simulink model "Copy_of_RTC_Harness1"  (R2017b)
settings: Solver=FixedStepDiscrete  StartTime=0.0  StopTime=4  FixedStep=0.01  RelTol=1e-3  EnableMultiTasking=on
undefined symbols (not defined in the file): sigbuilder_block

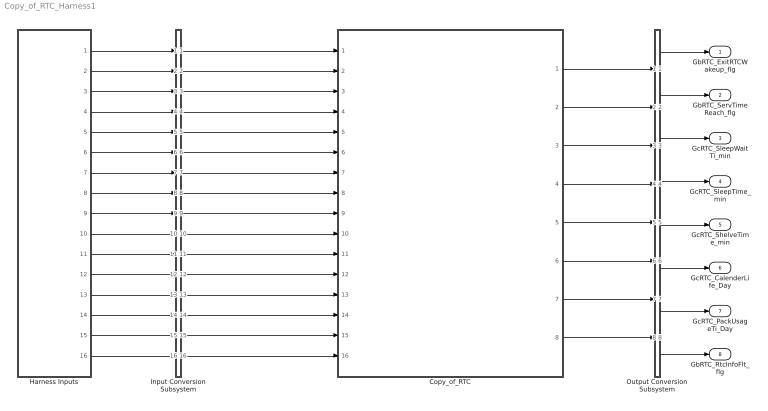
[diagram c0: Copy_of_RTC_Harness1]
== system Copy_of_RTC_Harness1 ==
  Copy_of_RTC : ModelReference  ModelNameDialog=Copy_of_RTC  SimulationMode=Normal  ModelReferenceVersion='M101C100'
  Harness Inputs : Subsystem  Tag=STV Subsys  LoadFcn=sigbuilder_block('load');  StartFcn=sigbuilder_block('start');  StopFcn=sigbuilder_block('stop');  ClipboardFcn=sigbuilder_block('clipboard');  mask(Sigbuilder block){tuvar=[0:10]}
      mask init:
      | if ~strcmp(get_param(bdroot(gcb),'SimulationStatus'),'stopped'),tuvar = sigbuilder_block('maskInit'); end
  Input Conversion Subsystem : Subsystem  Tag=__SLT_ICS__  Description=Signal spec. and routing
  Output Conversion Subsystem : Subsystem  Tag=__SLT_OCS__  Description=Signal spec. and routing
  GbRTC_ExitRTCWakeup_flg : Outport  OutDataTypeStr=boolean  PortDimensions=[1]
  GbRTC_ServTimeReach_flg : Outport  Port=2  OutDataTypeStr=boolean  PortDimensions=[1]
  GcRTC_SleepWaitTi_min : Outport  Port=3  OutDataTypeStr=uint16  PortDimensions=[1]
  GcRTC_SleepTime_min : Outport  Port=4  OutDataTypeStr=uint32  PortDimensions=[1]
  GcRTC_ShelveTime_min : Outport  Port=5  OutDataTypeStr=uint32  PortDimensions=[1]
  GcRTC_CalenderLife_Day : Outport  Port=6  OutDataTypeStr=uint32  PortDimensions=[1]
  GcRTC_PackUsageTi_Day : Outport  Port=7  OutDataTypeStr=uint32  PortDimensions=[1]
  GbRTC_RtcInfoFlt_flg : Outport  Port=8  OutDataTypeStr=boolean  PortDimensions=[1]
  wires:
  Harness Inputs/1(GbADP_RealTimeVld_flg) -> Input Conversion Subsystem/1(Inport_1)
  Harness Inputs/2(GbNDP_ReadShutdownTimeVld_flg) -> Input Conversion Subsystem/2(Inport_2)
  Harness Inputs/3(GcADP_YearSet_Yr) -> Input Conversion Subsystem/3(Inport_3)
  Harness Inputs/4(GcADP_MonthSet_Mn) -> Input Conversion Subsystem/4(Inport_4)
  Harness Inputs/5(GcADP_DaySet_D) -> Input Conversion Subsystem/5(Inport_5)
  Harness Inputs/6(GcADP_HourSet_Hr) -> Input Conversion Subsystem/6(Inport_6)
  Harness Inputs/7(GcADP_MinSet_Min) -> Input Conversion Subsystem/7(Inport_7)
  Harness Inputs/8(GcADP_SecondSet_S) -> Input Conversion Subsystem/8(Inport_8)
  Harness Inputs/9(GcISP_EcuOffTi_s) -> Input Conversion Subsystem/9(Inport_9)
  Harness Inputs/10(GeISP_EcuOffTiSt_enum) -> Input Conversion Subsystem/10(Inport_10)
  Harness Inputs/11(GeADP_AppChrgOrdCmd_enum) -> Input Conversion Subsystem/11(Inport_11)
  Harness Inputs/12(GeADP_AppChrgOrdStart_enum) -> Input Conversion Subsystem/12(Inport_12)
  Harness Inputs/13(GeMSM_BMUState_enum) -> Input Conversion Subsystem/13(Inport_13)
  Harness Inputs/14(GeODP_ObcCcSt_enum) -> Input Conversion Subsystem/14(Inport_14)
  Harness Inputs/15(GcADP_AcmDist_numb) -> Input Conversion Subsystem/15(Inport_15)
  Harness Inputs/16(GeCTC_CtrCtlState_enum) -> Input Conversion Subsystem/16(Inport_16)
  Output Conversion Subsystem/1(Outport_1) -> GbRTC_ExitRTCWakeup_flg/1
  Output Conversion Subsystem/2(Outport_2) -> GbRTC_ServTimeReach_flg/1
  Output Conversion Subsystem/3(Outport_3) -> GcRTC_SleepWaitTi_min/1
  Output Conversion Subsystem/4(Outport_4) -> GcRTC_SleepTime_min/1
  Output Conversion Subsystem/5(Outport_5) -> GcRTC_ShelveTime_min/1
  Output Conversion Subsystem/6(Outport_6) -> GcRTC_CalenderLife_Day/1
  Output Conversion Subsystem/7(Outport_7) -> GcRTC_PackUsageTi_Day/1
  Output Conversion Subsystem/8(Outport_8) -> GbRTC_RtcInfoFlt_flg/1
  Input Conversion Subsystem/1(Outport_1) -> Copy_of_RTC/1
  Input Conversion Subsystem/2(Outport_2) -> Copy_of_RTC/2
  Input Conversion Subsystem/3(Outport_3) -> Copy_of_RTC/3
  Input Conversion Subsystem/4(Outport_4) -> Copy_of_RTC/4
  Input Conversion Subsystem/5(Outport_5) -> Copy_of_RTC/5
  Input Conversion Subsystem/6(Outport_6) -> Copy_of_RTC/6
  Input Conversion Subsystem/7(Outport_7) -> Copy_of_RTC/7
  Input Conversion Subsystem/8(Outport_8) -> Copy_of_RTC/8
  Input Conversion Subsystem/9(Outport_9) -> Copy_of_RTC/9
  Input Conversion Subsystem/10(Outport_10) -> Copy_of_RTC/10
  Input Conversion Subsystem/11(Outport_11) -> Copy_of_RTC/11
  Input Conversion Subsystem/12(Outport_12) -> Copy_of_RTC/12
  Input Conversion Subsystem/13(Outport_13) -> Copy_of_RTC/13
  Input Conversion Subsystem/14(Outport_14) -> Copy_of_RTC/14
  Input Conversion Subsystem/15(Outport_15) -> Copy_of_RTC/15
  Input Conversion Subsystem/16(Outport_16) -> Copy_of_RTC/16
  Copy_of_RTC/1 -> Output Conversion Subsystem/1(Inport_1)
  Copy_of_RTC/2 -> Output Conversion Subsystem/2(Inport_2)
  Copy_of_RTC/3 -> Output Conversion Subsystem/3(Inport_3)
  Copy_of_RTC/4 -> Output Conversion Subsystem/4(Inport_4)
  Copy_of_RTC/5 -> Output Conversion Subsystem/5(Inport_5)
  Copy_of_RTC/6 -> Output Conversion Subsystem/6(Inport_6)
  Copy_of_RTC/7 -> Output Conversion Subsystem/7(Inport_7)
  Copy_of_RTC/8 -> Output Conversion Subsystem/8(Inport_8)

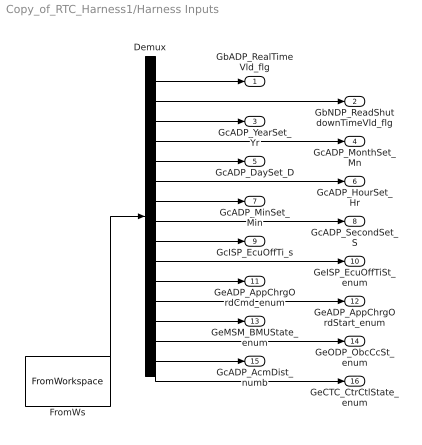
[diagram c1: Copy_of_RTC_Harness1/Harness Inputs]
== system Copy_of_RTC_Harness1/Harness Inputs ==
  Demux : Demux  Tag=STV Demux  Outputs=16
  FromWs : FromWorkspace  Tag=STV FromWs  VariableName=tuvar  SampleTime=0
  GbADP_RealTimeVld_flg : Outport  Tag=STV Outport
  GbNDP_ReadShutdownTimeVld_flg : Outport  Tag=STV Outport  Port=2
  GcADP_YearSet_Yr : Outport  Tag=STV Outport  Port=3
  GcADP_MonthSet_Mn : Outport  Tag=STV Outport  Port=4
  GcADP_DaySet_D : Outport  Tag=STV Outport  Port=5
  GcADP_HourSet_Hr : Outport  Tag=STV Outport  Port=6
  GcADP_MinSet_Min : Outport  Tag=STV Outport  Port=7
  GcADP_SecondSet_S : Outport  Tag=STV Outport  Port=8
  GcISP_EcuOffTi_s : Outport  Tag=STV Outport  Port=9
  GeISP_EcuOffTiSt_enum : Outport  Tag=STV Outport  Port=10
  GeADP_AppChrgOrdCmd_enum : Outport  Tag=STV Outport  Port=11
  GeADP_AppChrgOrdStart_enum : Outport  Tag=STV Outport  Port=12
  GeMSM_BMUState_enum : Outport  Tag=STV Outport  Port=13
  GeODP_ObcCcSt_enum : Outport  Tag=STV Outport  Port=14
  GcADP_AcmDist_numb : Outport  Tag=STV Outport  Port=15
  GeCTC_CtrCtlState_enum : Outport  Tag=STV Outport  Port=16
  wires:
  FromWs/1 -> Demux/1
  Demux/1 -> GbADP_RealTimeVld_flg/1
  Demux/2 -> GbNDP_ReadShutdownTimeVld_flg/1
  Demux/3 -> GcADP_YearSet_Yr/1
  Demux/4 -> GcADP_MonthSet_Mn/1
  Demux/5 -> GcADP_DaySet_D/1
  Demux/6 -> GcADP_HourSet_Hr/1
  Demux/7 -> GcADP_MinSet_Min/1
  Demux/8 -> GcADP_SecondSet_S/1
  Demux/9 -> GcISP_EcuOffTi_s/1
  Demux/10 -> GeISP_EcuOffTiSt_enum/1
  Demux/11 -> GeADP_AppChrgOrdCmd_enum/1
  Demux/12 -> GeADP_AppChrgOrdStart_enum/1
  Demux/13 -> GeMSM_BMUState_enum/1
  Demux/14 -> GeODP_ObcCcSt_enum/1
  Demux/15 -> GcADP_AcmDist_numb/1
  Demux/16 -> GeCTC_CtrCtlState_enum/1

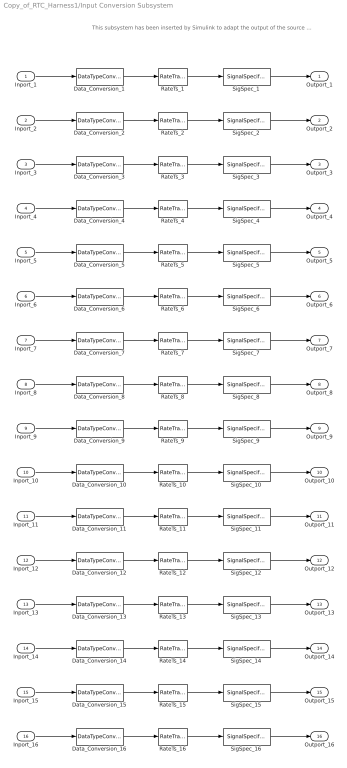
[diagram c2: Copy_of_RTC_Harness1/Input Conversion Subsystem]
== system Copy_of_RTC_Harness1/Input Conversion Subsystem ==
  note: This subsystem has been inserted by Simulink to adapt the output of the source blocks to the interface required by the harnessed component. Modifying the contents of this subsystem may result in compilation and simulation failure.
  Inport_1 : Inport
  Inport_2 : Inport  Port=2
  Inport_3 : Inport  Port=3
  Inport_4 : Inport  Port=4
  Inport_5 : Inport  Port=5
  Inport_6 : Inport  Port=6
  Inport_7 : Inport  Port=7
  Inport_8 : Inport  Port=8
  Inport_9 : Inport  Port=9
  Inport_10 : Inport  Port=10
  Inport_11 : Inport  Port=11
  Inport_12 : Inport  Port=12
  Inport_13 : Inport  Port=13
  Inport_14 : Inport  Port=14
  Inport_15 : Inport  Port=15
  Inport_16 : Inport  Port=16
  Data_Conversion_1 : DataTypeConversion  OutDataTypeStr=boolean
  Data_Conversion_{4..8,10..14,16} (11 alike) : DataTypeConversion  OutDataTypeStr=uint8
  Data_Conversion_15 : DataTypeConversion  OutDataTypeStr=single
  Data_Conversion_2 : DataTypeConversion  OutDataTypeStr=boolean
  Data_Conversion_3 : DataTypeConversion  OutDataTypeStr=uint16
  Data_Conversion_9 : DataTypeConversion  OutDataTypeStr=uint32
  RateTs_{1..16} (16 alike) : RateTransition  OutPortSampleTime=0.01
  SigSpec_1 : SignalSpecification  OutDataTypeStr=boolean  Unit=flg  Dimensions=[1]  SampleTime=0.01
  SigSpec_{10..13,16} (5 alike) : SignalSpecification  OutDataTypeStr=uint8  Unit=enum  Dimensions=[1]  SampleTime=0.01
  SigSpec_14 : SignalSpecification  OutDataTypeStr=uint8  Unit=numb  Dimensions=[1]  SampleTime=0.01
  SigSpec_15 : SignalSpecification  OutDataTypeStr=single  Unit=numb  Dimensions=[1]  SampleTime=0.01
  SigSpec_2 : SignalSpecification  OutDataTypeStr=boolean  Unit=flag  Dimensions=[1]  SampleTime=0.01
  SigSpec_3 : SignalSpecification  OutDataTypeStr=uint16  Unit=Yr  Dimensions=[1]  SampleTime=0.01
  SigSpec_4 : SignalSpecification  OutDataTypeStr=uint8  Unit=Min  Dimensions=[1]  SampleTime=0.01
  SigSpec_5 : SignalSpecification  OutDataTypeStr=uint8  Unit=Day  Dimensions=[1]  SampleTime=0.01
  SigSpec_6 : SignalSpecification  OutDataTypeStr=uint8  Unit=Hour  Dimensions=[1]  SampleTime=0.01
  SigSpec_7 : SignalSpecification  OutDataTypeStr=uint8  Unit=Min  Dimensions=[1]  SampleTime=0.01
  SigSpec_8 : SignalSpecification  OutDataTypeStr=uint8  Unit=S  Dimensions=[1]  SampleTime=0.01
  SigSpec_9 : SignalSpecification  OutDataTypeStr=uint32  Unit=s  Dimensions=[1]  SampleTime=0.01
  Outport_1 : Outport
  Outport_2 : Outport  Port=2
  Outport_3 : Outport  Port=3
  Outport_4 : Outport  Port=4
  Outport_5 : Outport  Port=5
  Outport_6 : Outport  Port=6
  Outport_7 : Outport  Port=7
  Outport_8 : Outport  Port=8
  Outport_9 : Outport  Port=9
  Outport_10 : Outport  Port=10
  Outport_11 : Outport  Port=11
  Outport_12 : Outport  Port=12
  Outport_13 : Outport  Port=13
  Outport_14 : Outport  Port=14
  Outport_15 : Outport  Port=15
  Outport_16 : Outport  Port=16
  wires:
  SigSpec_1/1 -> Outport_1/1
  RateTs_1/1 -> SigSpec_1/1
  Data_Conversion_1/1 -> RateTs_1/1
  Inport_1/1 -> Data_Conversion_1/1
  SigSpec_2/1 -> Outport_2/1
  RateTs_2/1 -> SigSpec_2/1
  Data_Conversion_2/1 -> RateTs_2/1
  Inport_2/1 -> Data_Conversion_2/1
  SigSpec_3/1 -> Outport_3/1
  RateTs_3/1 -> SigSpec_3/1
  Data_Conversion_3/1 -> RateTs_3/1
  Inport_3/1 -> Data_Conversion_3/1
  SigSpec_4/1 -> Outport_4/1
  RateTs_4/1 -> SigSpec_4/1
  Data_Conversion_4/1 -> RateTs_4/1
  Inport_4/1 -> Data_Conversion_4/1
  SigSpec_5/1 -> Outport_5/1
  RateTs_5/1 -> SigSpec_5/1
  Data_Conversion_5/1 -> RateTs_5/1
  Inport_5/1 -> Data_Conversion_5/1
  SigSpec_6/1 -> Outport_6/1
  RateTs_6/1 -> SigSpec_6/1
  Data_Conversion_6/1 -> RateTs_6/1
  Inport_6/1 -> Data_Conversion_6/1
  SigSpec_7/1 -> Outport_7/1
  RateTs_7/1 -> SigSpec_7/1
  Data_Conversion_7/1 -> RateTs_7/1
  Inport_7/1 -> Data_Conversion_7/1
  SigSpec_8/1 -> Outport_8/1
  RateTs_8/1 -> SigSpec_8/1
  Data_Conversion_8/1 -> RateTs_8/1
  Inport_8/1 -> Data_Conversion_8/1
  SigSpec_9/1 -> Outport_9/1
  RateTs_9/1 -> SigSpec_9/1
  Data_Conversion_9/1 -> RateTs_9/1
  Inport_9/1 -> Data_Conversion_9/1
  SigSpec_10/1 -> Outport_10/1
  RateTs_10/1 -> SigSpec_10/1
  Data_Conversion_10/1 -> RateTs_10/1
  Inport_10/1 -> Data_Conversion_10/1
  SigSpec_11/1 -> Outport_11/1
  RateTs_11/1 -> SigSpec_11/1
  Data_Conversion_11/1 -> RateTs_11/1
  Inport_11/1 -> Data_Conversion_11/1
  SigSpec_12/1 -> Outport_12/1
  RateTs_12/1 -> SigSpec_12/1
  Data_Conversion_12/1 -> RateTs_12/1
  Inport_12/1 -> Data_Conversion_12/1
  SigSpec_13/1 -> Outport_13/1
  RateTs_13/1 -> SigSpec_13/1
  Data_Conversion_13/1 -> RateTs_13/1
  Inport_13/1 -> Data_Conversion_13/1
  SigSpec_14/1 -> Outport_14/1
  RateTs_14/1 -> SigSpec_14/1
  Data_Conversion_14/1 -> RateTs_14/1
  Inport_14/1 -> Data_Conversion_14/1
  SigSpec_15/1 -> Outport_15/1
  RateTs_15/1 -> SigSpec_15/1
  Data_Conversion_15/1 -> RateTs_15/1
  Inport_15/1 -> Data_Conversion_15/1
  SigSpec_16/1 -> Outport_16/1
  RateTs_16/1 -> SigSpec_16/1
  Data_Conversion_16/1 -> RateTs_16/1
  Inport_16/1 -> Data_Conversion_16/1

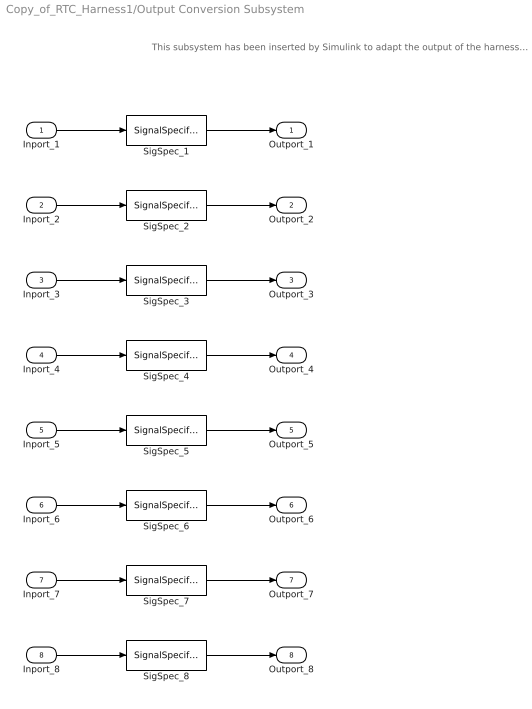
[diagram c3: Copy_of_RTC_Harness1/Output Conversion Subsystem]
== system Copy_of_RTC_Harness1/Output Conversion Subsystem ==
  note: This subsystem has been inserted by Simulink to adapt the output of the harnessed component to the interface required by the sink blocks. Modifying the contents of this subsystem may result in compilation and simulation failure.
  Inport_1 : Inport
  Inport_2 : Inport  Port=2
  Inport_3 : Inport  Port=3
  Inport_4 : Inport  Port=4
  Inport_5 : Inport  Port=5
  Inport_6 : Inport  Port=6
  Inport_7 : Inport  Port=7
  Inport_8 : Inport  Port=8
  SigSpec_1 : SignalSpecification  OutDataTypeStr=boolean  Unit=flg  Dimensions=[1]
  SigSpec_2 : SignalSpecification  OutDataTypeStr=boolean  Unit=flag  Dimensions=[1]
  SigSpec_3 : SignalSpecification  OutDataTypeStr=uint16  Unit=min  Dimensions=[1]
  SigSpec_4 : SignalSpecification  OutDataTypeStr=uint32  Unit=min  Dimensions=[1]  SampleTime=0.01
  SigSpec_5 : SignalSpecification  OutDataTypeStr=uint32  Unit=min  Dimensions=[1]  SampleTime=0.01
  SigSpec_6 : SignalSpecification  OutDataTypeStr=uint32  Unit=Day  Dimensions=[1]  SampleTime=0.01
  SigSpec_7 : SignalSpecification  OutDataTypeStr=uint32  Unit=Day  Dimensions=[1]  SampleTime=0.01
  SigSpec_8 : SignalSpecification  OutDataTypeStr=boolean  Unit=flag  Dimensions=[1]  SampleTime=0.01
  Outport_1 : Outport
  Outport_2 : Outport  Port=2
  Outport_3 : Outport  Port=3
  Outport_4 : Outport  Port=4
  Outport_5 : Outport  Port=5
  Outport_6 : Outport  Port=6
  Outport_7 : Outport  Port=7
  Outport_8 : Outport  Port=8
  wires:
  Inport_1/1 -> SigSpec_1/1
  SigSpec_1/1 -> Outport_1/1
  Inport_2/1 -> SigSpec_2/1
  SigSpec_2/1 -> Outport_2/1
  Inport_3/1 -> SigSpec_3/1
  SigSpec_3/1 -> Outport_3/1
  Inport_4/1 -> SigSpec_4/1
  SigSpec_4/1 -> Outport_4/1
  Inport_5/1 -> SigSpec_5/1
  SigSpec_5/1 -> Outport_5/1
  Inport_6/1 -> SigSpec_6/1
  SigSpec_6/1 -> Outport_6/1
  Inport_7/1 -> SigSpec_7/1
  SigSpec_7/1 -> Outport_7/1
  Inport_8/1 -> SigSpec_8/1
  SigSpec_8/1 -> Outport_8/1
